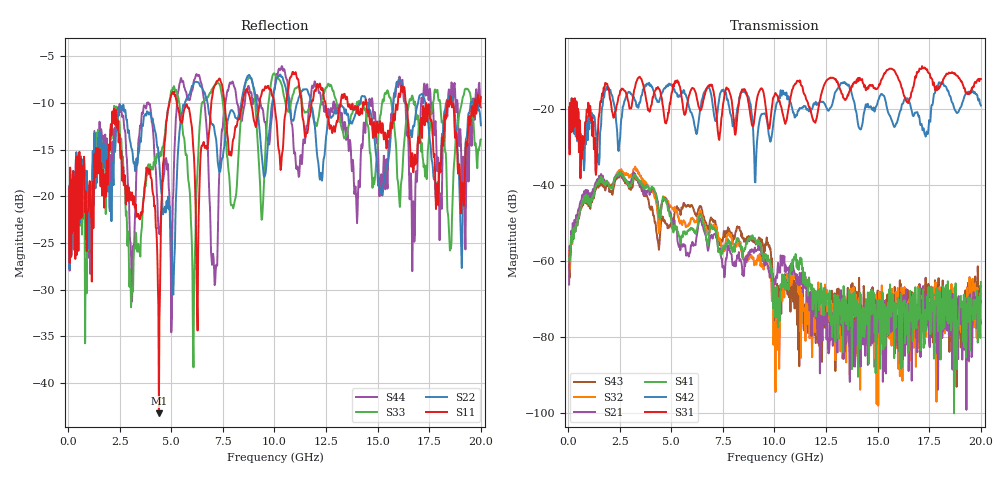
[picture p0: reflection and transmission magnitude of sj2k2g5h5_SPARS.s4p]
! FILE: E:\users\goganessyan\GBX_Backplane\FR408_backplane\1m_INBOUND_FEXT\sj2k2g5h5_SPARS.s4p
# MHZ S RI R 50.00
! FREQ  S11  S12  S13  S14
!  S21  S22  S23  S24
!  S31  S32  S33  S34
!  S41  S42  S43  S44
!  REAL  IMAG  REAL  IMAG  REAL  IMAG  REAL  IMAG
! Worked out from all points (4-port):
!   799 points, 50 MHz to 20 GHz, reference 50 ohm
!   strongest paths, dB at 50 MHz, 5.025 GHz, 10.03 GHz, 15.03 GHz, 20 GHz:
!     S31: -19.7, -15.7, -16.1, -14.5, -12.3
!     S42: -19.7, -14.0, -20.7, -17.8, -19.2
!     S41: -59.2, -50.5, -74.4, -75.0, -65.5
!     S21: -66.2, -49.4, -66.2, -73.1, -76.4
!     S32: -57.4, -45.9, -82.6, -98.0, -70.9
!     S43: -59.0, -50.4, -76.1, -87.3, -66.6
!   lowest |S11| = -43.2 dB at 4.4 GHz (marker M1), VSWR 1.01, Z = 50 + j0.687 ohm
!   |S11| at or under -10 dB: start of sweep to 4.91 GHz; 5.266 GHz to 6.94 GHz (1.674 GHz wide, 27.4 % of centre); 14.45 GHz to 15.98 GHz (1.527 GHz wide, 10 % of centre)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
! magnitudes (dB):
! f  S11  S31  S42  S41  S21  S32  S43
! 50 MHz  -19.1  -19.7  -19.7  -59.2  -66.2  -57.4  -59.0
! 1.6 GHz  -16.4  -18.3  -24.4  -37.9  -37.2  -37.8  -38.8
! 4.4 GHz  -43.2  -14.8  -18.3  -47.8  -46.6  -52.7  -57.1
! 5.075 GHz  -8.8  -14.8  -14.2  -50.9  -49.2  -46.3  -48.9
! 6.075 GHz  -15.1  -14.8  -22.8  -51.6  -56.1  -49.0  -46.3
! 10.03 GHz  -10.7  -16.1  -20.7  -74.4  -66.2  -82.6  -76.1
! 20 GHz  -9.4  -12.3  -19.2  -65.5  -76.4  -70.9  -66.6
